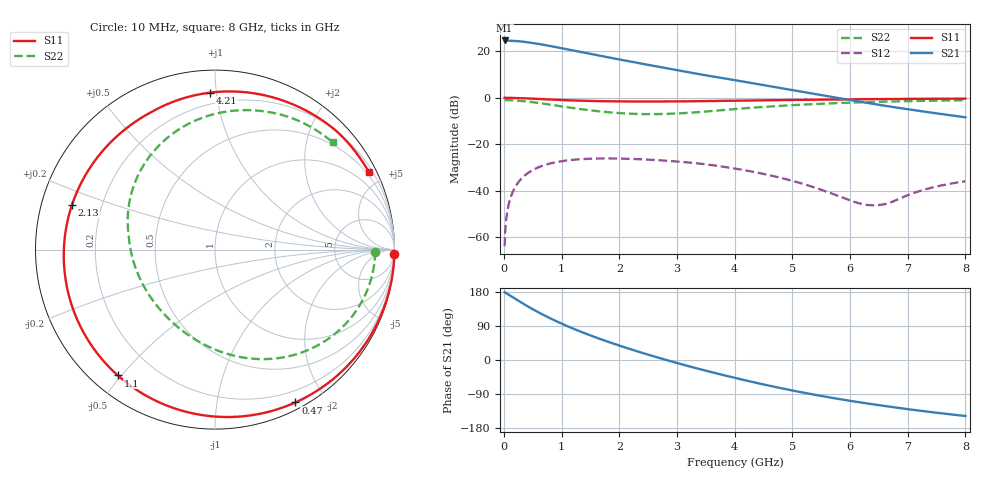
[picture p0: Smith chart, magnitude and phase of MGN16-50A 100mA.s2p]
! Port[1] = GATE
! Port[2] = DRAIN
! [Type]  S-parameter s2p file touchstone ver. 1.0
! [Object]  MGN16-50A
! [Bias]  100 mA
! [Version]  1.0
! [Date]  Thu May 28 10:54:03 2026
! [Source]  This file was created in JSC "ICC Milandr".
! [Disclaimer] Property of JSC "ICC Milandr". Unauthorized reproduction and/or distribution is strictly prohibited.
!  The file and the data are provided "AS IS" and with all faults and disclaim all warranties, express and implied, including
!  without limitation any implied warranties of merchantability, fitness for a particular purpose.
!  JSC "ICC Milandr" assumes no liability for:
!  1) the accuracy of the data provided;
!  2) the proper functioning of this data;
!  3) infringement of patents, copyrights or intellectual property rights resulting from the use of this data.
!  JSC "ICC Milandr" reserves the right to make changes to the products and the data without prior notice.
!  Please, be aware that your receipt and use of the file provided shall serve as acceptance of these terms and conditions.
!  If you do not accept these terms, you should return or destroy this file and any other accompanying information immediately.
# hz S ma R 12.5
! 2 Port Network Data from SP1.SP block
! freq  magS11  angS11  magS21  angS21  magS12  angS12  magS22  angS22
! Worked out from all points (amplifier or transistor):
!   800 points, 10 MHz to 8 GHz, reference 12.5 ohm
!   highest |S21| = 24.7 dB at 10 MHz (marker M1)
!   |S21| within 3 dB of that: start of sweep to 929.3 MHz
!   unconditionally stable (mu >= 1): 4.328 GHz to end of sweep
!   at 1.34 GHz: K = 0.18, MSG = 23.1 dB, |S12| = -26.4 dB
!   at 4.01 GHz: K = 0.84, MSG = 19.0 dB, |S12| = -30.5 dB
!   at 8 GHz: K = 1.26, MAG = 10.7 dB, |S12| = -35.9 dB
!   S11 on the Smith chart (normalised r, x): 10 MHz: 2, -84; 470 MHz: 0.07, -1.65; 1.1 GHz: 0.08, -0.49; 2.13 GHz: 0.09, +0.15; 4.21 GHz: 0.13, +0.96; 8 GHz: 0.38, +4.16
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1e7  0.9994 -1.4  17.19 178.9  0.0006394 82.3  0.8925 -0.8
4e7  0.9991 -5.6  17.14 176.1  0.002531 84.5  0.8919 -3.2
1.1e8  0.9969 -15.2  17.02 169.3  0.006907 79.1  0.8875 -8.8
2.1e8  0.9906 -28.9  16.71 159.8  0.01295 70.3  0.8746 -16.6
3.4e8  0.978 -46.0  16.1 147.8  0.02021 59.0  0.8481 -26.4
4.7e8  0.9622 -62.2  15.32 136.4  0.0266 48.1  0.8138 -35.8
6.1e8  0.9437 -78.7  14.38 124.7  0.03242 37.1  0.772 -45.2
7.5e8  0.9253 -94.0  13.4 113.8  0.03716 26.7  0.7285 -54.1
9.1e8  0.9059 -110.2  12.3 102.1  0.04138 15.7  0.6799 -63.7
1.1e9  0.8859 -127.7  11.06 89.1  0.04498 3.5  0.6267 -74.3
1.35e9  0.8654 -148.1  9.607 73.5  0.0479 -11.1  0.5668 -87.5
1.52e9  0.8549 -160.5  8.73 63.6  0.04898 -20.4  0.5333 -96.2
1.71e9  0.846 -173.1  7.853 53.1  0.0495 -30.2  0.5025 -105.9
1.91e9  0.8394 174.8  7.035 42.6  0.04944 -40.0  0.4776 -116.1
2.13e9  0.8349 162.8  6.244 31.5  0.04881 -50.3  0.4587 -127.5
2.68e9  0.8333 137.7  4.662 5.9  0.04535 -74.4  0.447 -156.4
3.27e9  0.8429 116.7  3.421 -19.1  0.03975 -98.2  0.4816 173.6
4.01e9  0.8684 96.6  2.394 -47.4  0.02991 -119.4  0.574 142.3
4.21e9  0.8751 91.7  2.171 -54.6  0.02707 -124.2  0.6003 134.7
5.34e9  0.9097 67.6  1.238 -90.4  0.01223 -141.1  0.7302 97.8
6.67e9  0.9445 45.2  0.654 -122.8  0.005345 -78.0  0.8314 65.8
8e9  0.9601 26.8  0.3808 -147.7  0.01601 -61.0  0.887 42.3
